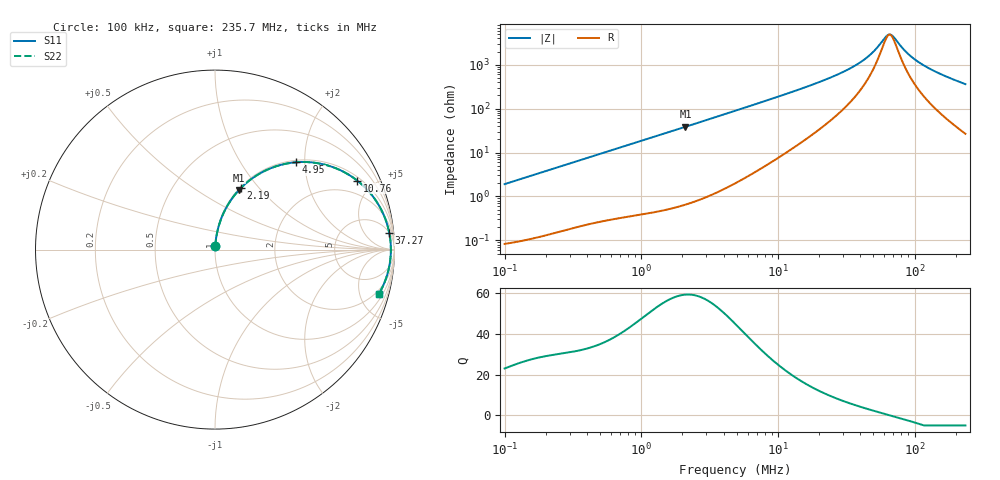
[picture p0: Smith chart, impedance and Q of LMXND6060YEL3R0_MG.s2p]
! LMXND6060YEL3R0_MG  S-PARAMETER MODEL  ( General Type )
! Model Generated by TAIYO YUDEN Corporation (http://www.ty-top.com)
! Version 1.0
! TAIYO YUDEN Control No. 191025NI43SB-FBB
! Copyright(c) 2019 TAIYO YUDEN CO.,LTD. All Rights Reserved.
! Product Description (link to TY-COMPAS)
! https://ds.yuden.co.jp/TYCOMPAS/or/detail?pn=LMXND6060YEL3R0NMG&u=M
! Products Name : Inductors
! Characteristics :
!  Inductance : 3.0 uH , SRF(min) : 45 MHz , DC Resistance(max) : 0.0312 Ohm
!  Rated Current : Saturation :5600 mA , Temp Rise : 3300 mA
!  Case Size : 6.0 x 6.0 / 0.236 x 0.236 [mm/inch] , Thickness : 4.5 / 0.177 [mm/inch]
!  (Conditions: Temperature = 25 degC , DC Bias Current/Voltage = 0A / 0V)
! External Node Assignments :
!  1  o---GGG---o  2
! GND o---------o GND
! Frequency Range : 0.1MHz  -  235.669543MHz  [ 402 STEP ]
# MHz S RI R 50
! Freq[MHz].  S11 Real  S11 Imag  S21 Real  S21 Imag  S12 Real  S12 Imag  S22 Real  S22 Imag
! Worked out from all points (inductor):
!   401 points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, 100 kHz to 235.7 MHz, reference 50 ohm
!   read as one part in series: L = 3.02 uH near 104 kHz
!   highest Q = 59.4 at 2.107 MHz (marker M1), where L = 2.91 uH
!   self-resonance near 65.73 MHz
!   S11 on the Smith chart (normalised r, x): 100 kHz: 1.00, +0.04; 2.19 MHz: 1.01, +0.80; 4.95 MHz: 1.04, +1.82; 10.76 MHz: 1.17, +4.03; 37.27 MHz: 5, +19; 235.7 MHz: 1.53, -7.21
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0.1  0.00119 0.019  0.9988 -0.019  0.9988 -0.019  0.00119 0.019
0.367165  0.00676 0.0678  0.9932 -0.0678  0.9932 -0.0678  0.00676 0.0678
0.73853  0.0213 0.1326  0.9787 -0.1326  0.9787 -0.1326  0.0213 0.1326
1.348099  0.0612 0.2306  0.9388 -0.2306  0.9388 -0.2306  0.0612 0.2306
2.106828  0.1334 0.3316  0.8666 -0.3316  0.8666 -0.3316  0.1334 0.3316
2.190235  0.1424 0.3411  0.8576 -0.3411  0.8576 -0.3411  0.1424 0.3411
3.167197  0.2551 0.4271  0.7449 -0.4271  0.7449 -0.4271  0.2551 0.4271
4.854581  0.4435 0.4858  0.5565 -0.4858  0.5565 -0.4858  0.4435 0.4858
4.949741  0.453 0.4867  0.547 -0.4867  0.547 -0.4867  0.453 0.4867
7.019984  0.623 0.4702  0.377 -0.4702  0.377 -0.4702  0.623 0.4702
10.76001  0.7924 0.3847  0.2076 -0.3847  0.2076 -0.3847  0.7924 0.3847
17.8243  0.9089 0.2537  0.0911 -0.2537  0.0911 -0.2537  0.9089 0.2537
27.32054  0.9546 0.1552  0.0454 -0.1552  0.0454 -0.1552  0.9546 0.1552
37.27189  0.9707 0.0949  0.0293 -0.0949  0.0293 -0.0949  0.9707 0.0949
47.04901  0.9769 0.0544  0.0231 -0.0544  0.0231 -0.0544  0.9769 0.0544
61.74206  0.9799 0.01  0.0201 -0.01  0.0201 -0.01  0.9799 0.01
65.44454  0.98 0.000673  0.02 -0.000673  0.02 -0.000673  0.98 0.000673
70.72882  0.9798 -0.0118  0.0202 0.0118  0.0202 0.0118  0.9798 -0.0118
91.03246  0.9771 -0.053  0.0229 0.053  0.0229 0.053  0.9771 -0.053
110.536  0.9723 -0.0864  0.0277 0.0864  0.0277 0.0864  0.9723 -0.0864
153.7541  0.9566 -0.1495  0.0434 0.1495  0.0434 0.1495  0.9566 -0.1495
235.6695  0.9132 -0.2469  0.0868 0.2469  0.0868 0.2469  0.9132 -0.2469
